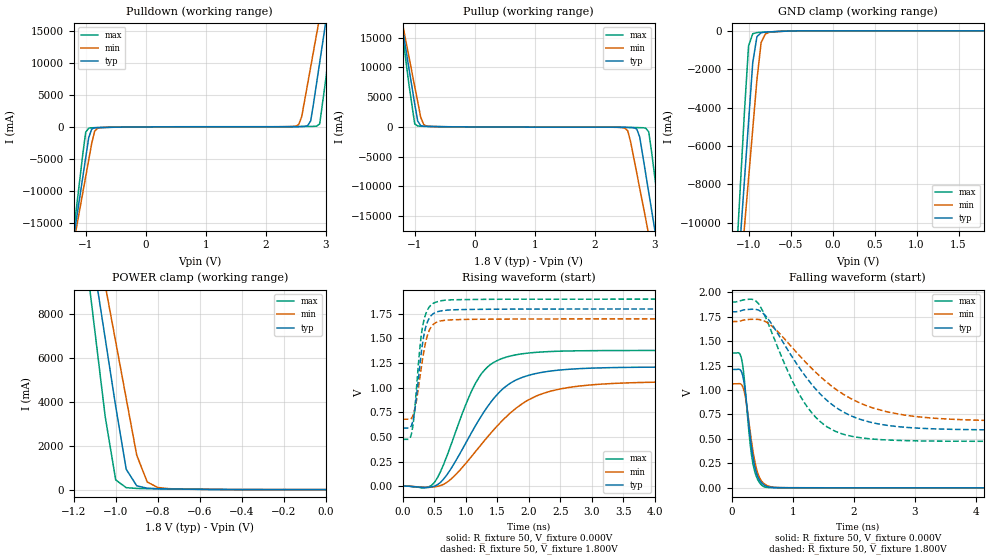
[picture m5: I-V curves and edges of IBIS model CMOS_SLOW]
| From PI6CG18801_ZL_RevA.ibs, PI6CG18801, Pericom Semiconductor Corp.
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[Model]   CMOS_SLOW
Model_type Output
Vref=1.800V
Vmeas=900mV
| variable   typ   min   max
C_comp   1.500pF   1.470pF   1.530pF
[Voltage Range]   1.8000V   1.7000V   1.9000V
[POWER Clamp Reference]   1.8000V   1.7000V   1.9000V
[GND Clamp Reference]   0.0000V   0.0000V   0.0000V
[Pullup Reference]   1.8000V   1.7000V   1.9000V
[Pulldown Reference]   0.0000V   0.0000V   0.0000V
[Temperature Range]   25   85   -40
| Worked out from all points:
|   slope of the pulldown table from 0 to 0.27 V, typ, clamps not added: 17.5 ohm
|   slope of the pullup table from 0 to 0.27 V, typ, clamps not added: 20 ohm
|   GND clamp passes 1 mA (typ) near -0.36 V on its own axis
|   POWER clamp passes 1 mA (typ) near -0.39 V on its own axis
|   falling waveform, R_fixture 50, V_fixture 0.000V: 20-80 % time 144ps typ, 155ps min, 132ps max; typ from 1.21 V to 0 V
|   rising waveform, R_fixture 50, V_fixture 0.000V: 20-80 % time 728ps typ, 954ps min, 527ps max; typ from 0 V to 1.21 V
|   falling waveform, R_fixture 50, V_fixture 1.800V: 20-80 % time 912ps typ, 1.14ns min, 682ps max; typ from 1.8 V to 0.59 V
|   rising waveform, R_fixture 50, V_fixture 1.800V: 20-80 % time 140ps typ, 156ps min, 127ps max; typ from 0.59 V to 1.8 V
[GND Clamp]
| Voltage   I(typ)   I(min)   I(max)
-1.8V     -54.4A     -49.03A    -63.81A
-1.15V    -14.07A    -15.45A    -12.25A
-1.1V     -10.96A    -12.87A    -8.279A
-1.05V    -7.862A    -10.28A    -4.312A
-1V       -4.76A     -7.701A    -788.1mA
-950mV    -1.658A    -5.119A    -151.5mA
-900mV    -302.5mA   -2.537A    -89.47mA
-850mV    -100.7mA   -612.3mA   -76.41mA
-800mV    -66.15mA   -166.6mA   -67.68mA
-750mV    -54.39mA   -72.37mA   -57.6mA
-350mV    -594.7uA   -1.401mA   -102.1uA
1.8V      15.03uA    16.7uA     13.92uA
[Power Clamp]
| Voltage   I(typ)   I(min)   I(max)
-1.8V     53.55A     48.18A     62.95A
-1.15V    13.11A     14.51A     11.28A
-1.1V     10.01A     11.92A     7.303A
-1.05V    6.9A       9.334A     3.331A
-1V       3.793A     6.748A     443mA
-950mV    928.9mA    4.161A     88.83mA
-900mV    175.4mA    1.576A     52.93mA
-850mV    61.99mA    347.9mA    44.07mA
-800mV    40.66mA    98.73mA    37.38mA
-750mV    32.05mA    44.28mA    30.27mA
-650mV    19.3mA     21.1mA     16.82mA
0V        15.03uA    14.98uA    14.69uA
[Pulldown]
| Voltage   I(typ)   I(min)   I(max)
-1.8V     -54.42A    -49.05A    -63.84A
-1.2V     -17.2A     -18.06A    -16.25A
-1V       -4.79A     -7.726A    -827.2mA
-950mV    -1.689A    -5.144A    -191.1mA
-750mV    -87.68mA   -99.6mA    -100.8mA
2.55V     59.88mA    370.4mA    52.99mA
2.75V     956.7mA    9.357A     80.67mA
2.85V     6.928A     14.53A     125.7mA
2.9V      10.03A     17.12A     480mA
3V        16.25A     22.3A      7.34A
3.1V      22.47A     27.48A     15.29A
3.6V      53.58A     53.39A     55.04A
[Pullup]
| Voltage   I(typ)   I(min)   I(max)
-1.8V     53.63A     48.25A     63.06A
-1.2V     16.29A     17.15A     15.33A
-1V       3.851A     6.797A     513.7mA
-950mV    984.1mA    4.208A     156.8mA
-800mV    86.58mA    137.9mA    94.43mA
2.5V      -78.71mA   -194.9mA   -67.08mA
2.7V      -336.9mA   -7.729A    -111.4mA
2.85V     -7.897A    -15.48A    -195.5mA
2.9V      -11A       -18.06A    -832.2mA
3V        -17.2A     -23.23A    -8.323A
3.1V      -23.41A    -28.39A    -16.26A
3.6V      -54.44A    -54.22A    -55.93A
[Falling Waveform]
R_fixture = 50
V_fixture = 0.000V
V_fixture_min = 0.000V
V_fixture_max = 0.000V
|   Time   V(typ)   V(min)   V(max)
0s        1.211V     1.064V     1.378V
120ps     1.212V     1.065V     1.378V
156ps     1.191V     1.058V     1.33V
192ps     1.111V     1.013V     1.194V
228ps     950.4mV    910.3mV    958.9mV
300ps     537.1mV    583.9mV    459.8mV
348ps     312.9mV    374.9mV    245.3mV
444ps     91.33mV    118.9mV    63.53mV
576ps     14.89mV    24.98mV    4.852mV
20ns      8.604uV    9.507uV    8.114uV
[Rising Waveform]
R_fixture = 50
V_fixture = 0.000V
V_fixture_min = 0.000V
V_fixture_max = 0.000V
|   Time   V(typ)   V(min)   V(max)
0s        8.589uV    9.475uV    8.119uV
500ps     -1.428mV   -8.049mV   34.32mV
750ps     160.3mV    62.23mV    390.2mV
1.05ns    494.9mV    268.7mV    904.2mV
1.25ns    714.6mV    425.4mV    1.143V
1.6ns     995.4mV    678.1mV    1.301V
2ns       1.126V     877.5mV    1.352V
2.65ns    1.188V     1.004V     1.373V
4ns       1.209V     1.056V     1.378V
20ns      1.211V     1.064V     1.378V
[Falling Waveform]
R_fixture = 50
V_fixture = 1.800V
V_fixture_min = 1.700V
V_fixture_max = 1.900V
|   Time   V(typ)   V(min)   V(max)
0s        1.8V       1.7V       1.9V
437.5ps   1.818V     1.722V     1.883V
625ps     1.701V     1.67V      1.637V
1ns       1.329V     1.427V     1.083V
1.375ns   1.01V      1.182V     721.4mV
1.688ns   830.4mV    1.016V     580.4mV
2.188ns   685.3mV    844.5mV    506mV
3ns       612.3mV    730mV      480.8mV
4.375ns   592.5mV    687.2mV    475.6mV
20ns      589.8mV    679.5mV    475mV
[Rising Waveform]
R_fixture = 50
V_fixture = 1.800V
V_fixture_min = 1.700V
V_fixture_max = 1.900V
|   Time   V(typ)   V(min)   V(max)
0s        589.8mV    679.5mV    475mV
110ps     592.2mV    679.7mV    484.1mV
150ps     635.8mV    700.1mV    566.4mV
200ps     813.8mV    806.8mV    851.8mV
290ps     1.328V     1.18V      1.51V
350ps     1.577V     1.417V     1.718V
390ps     1.664V     1.528V     1.786V
460ps     1.738V     1.625V     1.846V
660ps     1.785V     1.684V     1.888V
20ns      1.8V       1.7V       1.9V
[Ramp]
| variable   typ   min   max
dV/dt_r   0.72588V/726.77p   0.63570V/852.83p   0.82704V/522.78p
dV/dt_f   0.72584V/910.56p   0.61212V/1.1397n   1.00548V/678.01p
R_load = 50
